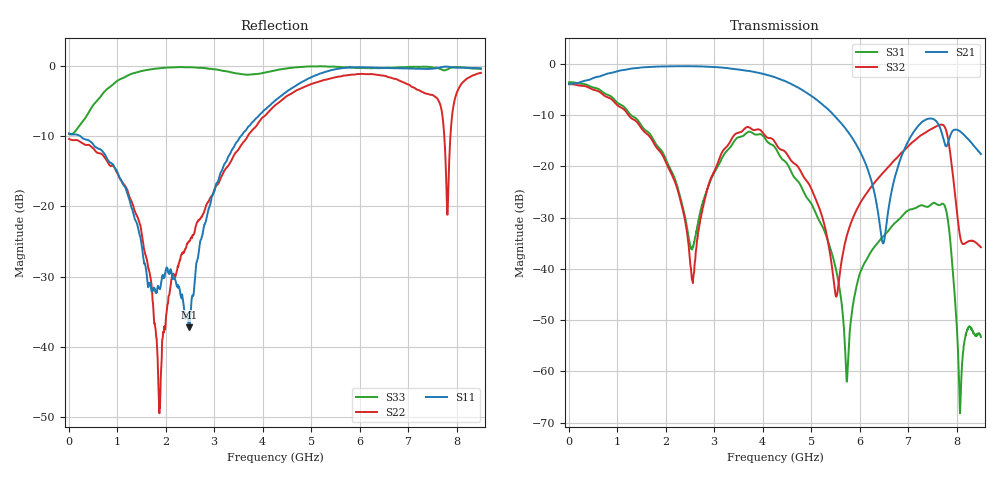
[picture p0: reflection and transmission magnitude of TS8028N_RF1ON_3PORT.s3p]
!Created with skrf (http://scikit-rf.org).
# GHz S RI R 50.0
!freq ReS11 ImS11 ReS12 ImS12 ReS13 ImS13
! ReS21 ImS21 ReS22 ImS22 ReS23 ImS23
! ReS31 ImS31 ReS32 ImS32 ReS33 ImS33
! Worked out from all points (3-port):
!   1601 points, 10 MHz to 8.5 GHz, reference 50 ohm
!   strongest paths, dB at 10 MHz, 2.132 GHz, 4.255 GHz, 6.378 GHz, 8.5 GHz:
!     S21: -3.9, -0.4, -2.6, -28.8, -17.6
!     S32: -3.9, -21.7, -15.3, -22.4, -35.8
!     S31: -3.6, -21.2, -16.3, -34.8, -53.3
!   lowest |S11| = -37.2 dB at 2.483 GHz (marker M1), VSWR 1.03, Z = 48.8 + j0.718 ohm
!   |S11| at or under -10 dB: 242.1 MHz to 3.55 GHz (3.308 GHz wide, 174 % of centre)
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0.01  -0.3304 0.0104  0.6393 0.00294  0.6642 -0.00932
      0.6392 0.00287  -0.3014 0.00933  0.6344 -0.00841
      0.6641 -0.00943  0.6346 -0.00828  -0.3265 0.0215
1.872494  0.00654 -0.0253  0.5925 -0.7353  -0.1343 -0.0672
          0.5924 -0.7353  -0.00331 0.000594  -0.1168 -0.0797
          -0.1342 -0.0669  -0.1168 -0.0799  0.2598 -0.9269
2.482712  -0.0117 0.00735  0.2491 -0.9181  -0.0162 -0.01
          0.2491 -0.9184  -0.00752 -0.056  -0.0141 0.00623
          -0.0162 -0.01  -0.014 0.00627  -0.3842 -0.9002
3.294569  0.0482 0.2215  -0.2984 -0.8599  -0.000851 -0.1471
          -0.2983 -0.8594  -0.1196 -0.1546  0.1175 -0.1138
          -0.000549 -0.1469  0.1177 -0.1136  -0.8837 0.2168
4.255  0.4735 0.3088  -0.6767 -0.3074  -0.1328 0.0774
       -0.6762 -0.3063  -0.5116 -0.1086  -0.1556 -0.0744
       -0.1327 0.0771  -0.1559 -0.0744  0.9212 0.1126
5.735444  0.8818 -0.4065  -0.1439 0.1741  0.000668 -0.000434
          -0.1437 0.1742  -0.1339 0.8475  0.00176 -0.021
          0.00067 -0.000423  0.00178 -0.021  0.4546 -0.865
6.483625  0.7162 -0.6503  -0.0177 -0.000623  -0.0183 -0.00968
          -0.0177 -0.000551  0.508 0.6843  -0.0256 -0.0831
          -0.0183 -0.00957  -0.0255 -0.0832  0.2086 -0.942
7.322012  0.5911 -0.7442  -0.2645 -0.0868  -0.0294 0.0289
          -0.2645 -0.0875  0.0459 -0.6424  -0.209 -0.00256
          -0.0294 0.0289  -0.2087 -0.00226  0.0994 -0.9824
8.070194  0.4933 -0.8373  -0.1702 0.1381  0.000244 0.000281
          -0.1711 0.1383  -0.6439 0.316  0.0159 0.0136
          0.000236 0.00031  0.0158 0.0135  0.1272 -0.9698
8.5  0.4541 -0.8481  -0.0533 0.1208  -0.00148 0.00165
     -0.0528 0.121  -0.2249 0.8634  0.000627 0.0163
     -0.00147 0.0016  0.000548 0.0163  0.04 -0.9506
